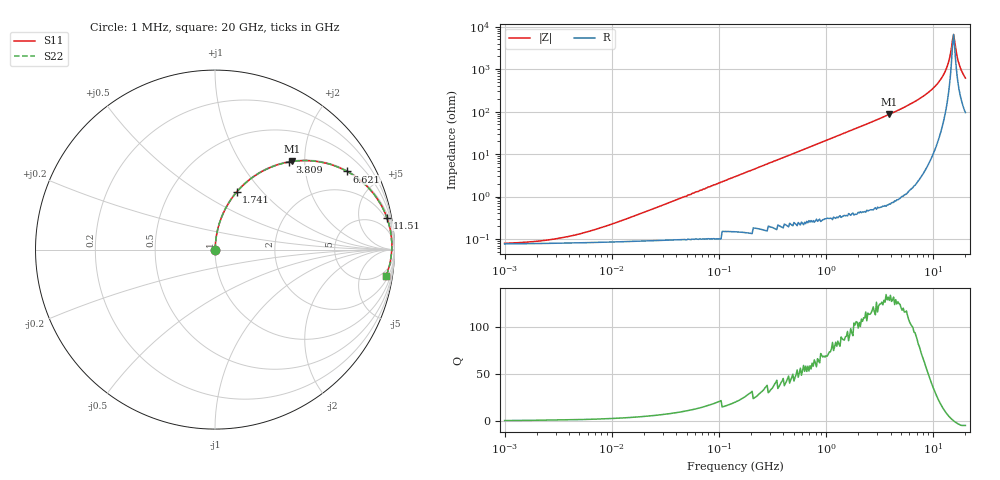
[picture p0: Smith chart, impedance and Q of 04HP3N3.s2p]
# MHz S MA R 50
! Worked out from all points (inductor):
!   431 points, 1 MHz to 20 GHz, reference 50 ohm
!   read as one part in series: L = 3.3 nH near 12.6 MHz
!   highest Q = 129 at 3.898 GHz (marker M1), where L = 3.52 nH
!   self-resonance near 15.17 GHz
!   S11 on the Smith chart (normalised r, x): 1 MHz: 1.00, +0.00; 1.741 GHz: 1.01, +0.73; 3.809 GHz: 1.01, +1.68; 6.621 GHz: 1.04, +3.36; 11.51 GHz: 2, +11; 20 GHz: 3, -12
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1  0.000567 21.4  0.999 -0.0  0.999 -0.0  0.000567 21.4
2.345  0.0007483 40.5  0.999 -0.0  0.999 -0.0  0.0007483 40.5
5.25  0.001256 59.9  0.999 -0.1  0.999 -0.1  0.001256 59.9
27.564  0.005775 81.1  0.999 -0.3  0.999 -0.3  0.005775 81.1
144.716  0.03 85.6  0.998 -1.7  0.998 -1.7  0.03 85.6
742.485  0.152 80.3  0.986 -8.8  0.986 -8.8  0.152 80.3
1740.909  0.342 69.4  0.936 -20.0  0.936 -20.0  0.342 69.4
2575.235  0.48 60.8  0.873 -28.7  0.873 -28.7  0.48 60.8
3809.408  0.641 49.7  0.763 -39.9  0.763 -39.9  0.641 49.7
3898.162  0.651 49.0  0.754 -40.6  0.754 -40.6  0.651 49.0
6620.869  0.855 30.6  0.509 -58.8  0.509 -58.8  0.855 30.6
9140.05  0.94 18.9  0.323 -69.9  0.323 -69.9  0.94 18.9
11507.27  0.974 10.6  0.183 -76.6  0.183 -76.6  0.974 10.6
13212.56  0.984 5.6  0.099 -77.6  0.099 -77.6  0.984 5.6
14157.74  0.985 3.2  0.057 -73.6  0.057 -73.6  0.985 3.2
14825.14  0.986 1.6  0.031 -61.2  0.031 -61.2  0.986 1.6
15524  0.985 -0.0  0.015 2.8  0.015 2.8  0.985 -0.0
15885.69  0.984 -0.8  0.022 42.1  0.022 42.1  0.984 -0.8
17022.1  0.98 -3.3  0.06 69.2  0.06 69.2  0.98 -3.3
17824.53  0.977 -4.9  0.087 72.2  0.087 72.2  0.977 -4.9
19099.64  0.97 -7.3  0.128 72.8  0.128 72.8  0.97 -7.3
20000  0.964 -8.8  0.156 72.3  0.156 72.3  0.964 -8.8
